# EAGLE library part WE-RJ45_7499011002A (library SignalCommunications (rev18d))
Order Code 7499011002A Design THT xBase-T 10/100 Base-T Ports 1x1 Application Standard Tab Position Down LED (Left-Right) NONE EMI Fingers Yes Details see: http://katalog.we-online.de/en/pbs/WE-LAN_RJ45/7499010001A? Updated by Yingchun Shan 2016-08-29 2016(C) Würth Elektronik
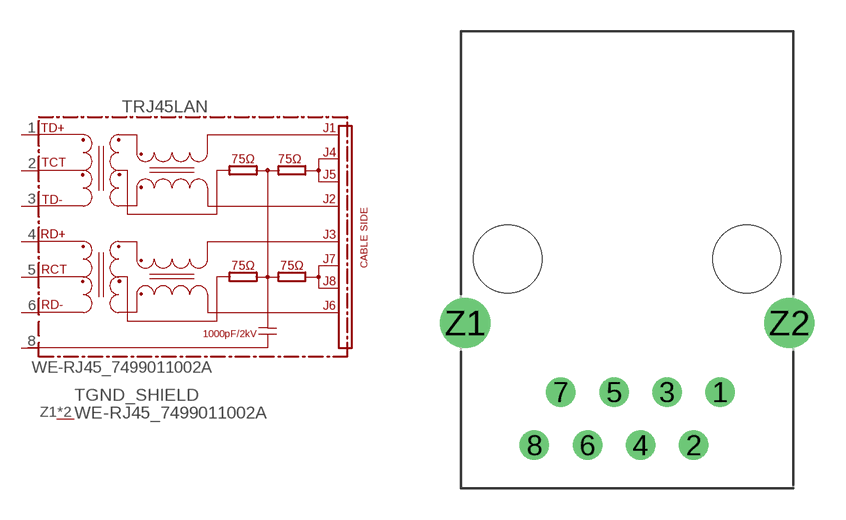
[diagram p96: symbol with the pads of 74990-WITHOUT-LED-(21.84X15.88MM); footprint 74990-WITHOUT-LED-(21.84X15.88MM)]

Designator prefix T; gates RJ45LAN=74990X-THT-10/100-T GND_SHIELD=GND_PIN

## WE-RJ45_7499011002A (COMPANY-URL: http://www.we-online.de; CREATED-BY: Christin Zierenner; CREATED-DATE: AUG 2012; DATASHEET-URL: http://katalog.we-online.de/kataloge/eisos/media/pdf/7499011002A.pdf; MANUFACTURER: Würth Elektronik eiSos GmbH)  [74990-WITHOUT-LED-(21.84X15.88MM)]
1  RJ45LAN:TD+
2  RJ45LAN:TCT
3  RJ45LAN:TD-
4  RJ45LAN:RD+
5  RJ45LAN:RCT
6  RJ45LAN:RD-
8  RJ45LAN:8
Z1  GND_SHIELD:1  pwr
Z2  GND_SHIELD:1  pwr

## Footprint 74990-WITHOUT-LED-(21.84X15.88MM) (pad centres in mm)
MAX HEIGHT=13.95mm PORTS----1X1 LED ----NO
drill 0.9: 1 4.445,-6.35; 2 3.175,-8.89; 3 1.905,-6.35; 4 0.635,-8.89; 5 -0.635,-6.35; 6 -1.905,-8.89; 7 -3.175,-6.35; 8 -4.445,-8.89
drill 1.6: Z1 -7.745,-3.05; Z2 7.745,-3.05
hole 3.25 at 5.715,0
hole 3.25 at -5.715,0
